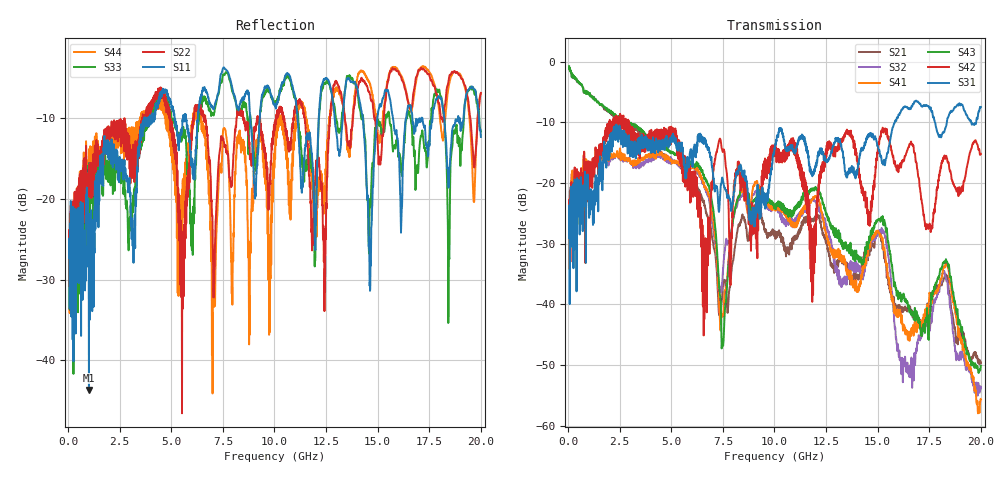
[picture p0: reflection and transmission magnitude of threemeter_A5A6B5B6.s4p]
! FILE: D:\iPass\iPassCable1005\iPassCable\SOLT_cal\threemeter_A5A6B5B6.s4p
# MHz S MA R 50.00
! FREQ  S11  S12  S13  S14
!  S21  S22  S23  S24
!  S31  S32  S33  S34
!  S41  S42  S43  S44
!  MAG  ANG  MAG  ANG  MAG  ANG  MAG  ANG
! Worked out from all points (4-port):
!   1996 points, 50 MHz to 20 GHz, reference 50 ohm
!   strongest paths, dB at 50 MHz, 5.04 GHz, 10.03 GHz, 15.02 GHz, 20 GHz:
!     S31: -29.0, -12.2, -13.9, -14.2, -7.5
!     S42: -27.8, -11.0, -14.9, -14.2, -15.2
!     S43: -0.7, -15.0, -23.7, -26.0, -50.1
!     S41: -25.5, -16.7, -23.9, -27.9, -55.6
!     S32: -25.5, -16.3, -23.7, -28.1, -53.8
!     S21: -0.8, -16.1, -27.9, -27.9, -49.7
!   lowest |S11| = -43.7 dB at 1.01 GHz (marker M1), VSWR 1.01, Z = 49.5 + j0.351 ohm
!   |S11| at or under -10 dB: start of sweep to 3.698 GHz; 11.11 GHz to 12.14 GHz (1.029 GHz wide, 8.85 % of centre); 14.28 GHz to 14.98 GHz (705.1 MHz wide, 4.82 % of centre)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
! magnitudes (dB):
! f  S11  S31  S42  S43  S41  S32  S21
! 50 MHz  -27.3  -29.0  -27.8  -0.7  -25.5  -25.5  -0.8
! 1.01 GHz  -43.7  -24.1  -18.1  -5.3  -17.7  -18.0  -5.3
! 6.47 GHz  -7.3  -12.3  -26.0  -17.9  -19.2  -19.2  -22.3
! 7.05 GHz  -8.9  -19.2  -17.8  -24.7  -26.7  -28.1  -30.4
! 7.5 GHz  -3.9  -19.6  -14.8  -46.8  -42.0  -34.6  -37.0
! 12.03 GHz  -19.8  -17.2  -26.1  -20.8  -22.1  -23.3  -25.3
! 20 GHz  -12.4  -7.5  -15.2  -50.1  -55.6  -53.8  -49.7
